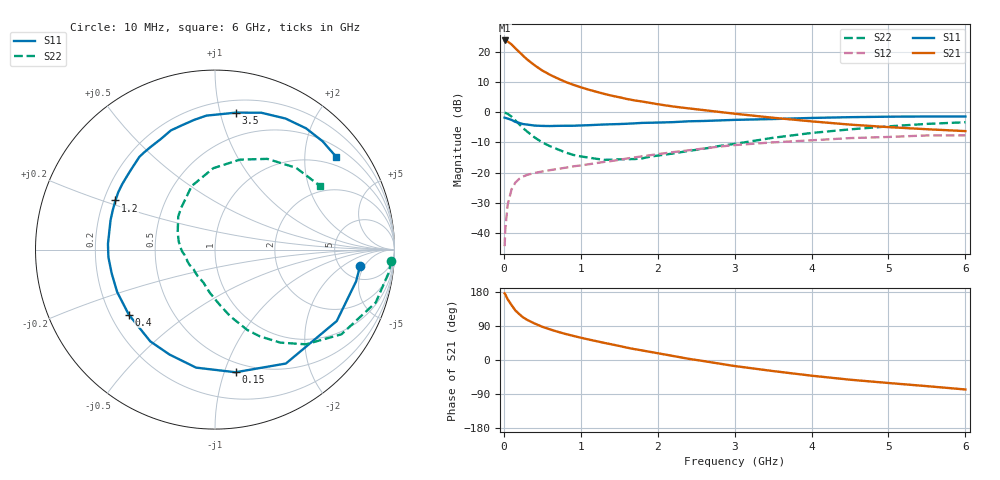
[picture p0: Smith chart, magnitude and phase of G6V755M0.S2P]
! SIEMENS Small Signal Semiconductors
! BFG193
! Si NPN RF Bipolar Junction Transistor in SOT223
! VCE = 0.75 V  IC = 5 mA
! Common Emitter S-Parameters:  August  1996
# GHz  S  MA  R  50
!  f  S11  S21  S12  S22
! GHz  MAG  ANG  MAG  ANG  MAG  ANG  MAG  ANG
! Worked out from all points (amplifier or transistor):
!   36 points, 10 MHz to 6 GHz, reference 50 ohm
!   highest |S21| = 23.8 dB at 10 MHz (marker M1)
!   |S21| within 3 dB of that: start of sweep to 165.9 MHz
!   unconditionally stable (mu >= 1): 1.043 GHz to 3.65 GHz
!   at 250 MHz: K = 0.35, MSG = 20.0 dB, |S12| = -21.3 dB
!   at 1.4 GHz: K = 1.10, MAG = 8.9 dB, |S12| = -16.2 dB
!   at 6 GHz: K = 0.99, MSG = 0.7 dB, |S12| = -7.7 dB
!   S11 on the Smith chart (normalised r, x): 10 MHz: 7.47, -4.06; 150 MHz: 0.42, -1.09; 400 MHz: 0.27, -0.31; 1.2 GHz: 0.25, +0.22; 3.5 GHz: 0.30, +1.12; 6 GHz: 0.75, +2.78
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0.01  0.8133 -6.5  15.55 175.9  0.006 89.4  0.9839 -3.6
0.02  0.8058 -12.7  15.46 172.8  0.012 84.6  0.9773 -7.4
0.05  0.7865 -30.4  14.94 160.2  0.0294 73.9  0.9429 -18.2
0.1  0.7476 -58.1  13.4 144.9  0.0525 62.4  0.848 -33.8
0.15  0.6929 -80.5  11.5 130.8  0.0682 51.8  0.7312 -46.2
0.2  0.666 -99.1  10.02 121.1  0.0786 45.5  0.6336 -54.9
0.25  0.6373 -113.4  8.661 112.6  0.0858 40.7  0.5447 -62.6
0.3  0.6257 -125.2  7.581 106.2  0.0911 37.7  0.4828 -68.1
0.4  0.6015 -143.0  6.021 96.3  0.0986 33.9  0.3824 -77.0
0.5  0.5941 -156.6  4.929 87.6  0.104 31.6  0.3158 -84.2
0.6  0.5907 -167.0  4.191 80.8  0.1095 30.9  0.2737 -90.4
0.7  0.5954 -175.9  3.645 74.5  0.1146 30.6  0.2428 -96.7
0.9  0.5973 170.5  2.871 63.7  0.1264 30.4  0.1964 -108.6
1.1  0.6101 159.2  2.377 54.2  0.1369 30.0  0.1772 -122.4
1.2  0.6186 153.7  2.193 49.8  0.1432 30.1  0.1693 -129.4
1.6  0.6454 136.7  1.66 32.6  0.171 27.6  0.1667 -156.9
2.2  0.6858 116.2  1.247 10.6  0.2178 20.6  0.2069 167.5
2.8  0.7324 99.0  1.013 -9.5  0.2695 10.4  0.276 137.9
3.5  0.7721 81.3  0.811 -29.2  0.3168 -4.9  0.3774 110.1
4.5  0.8293 61.7  0.624 -52.0  0.3728 -24.0  0.5203 74.5
5.5  0.8506 45.2  0.523 -69.0  0.4127 -46.9  0.6417 45.2
6  0.8505 37.3  0.487 -77.8  0.4136 -60.0  0.6832 31.5
